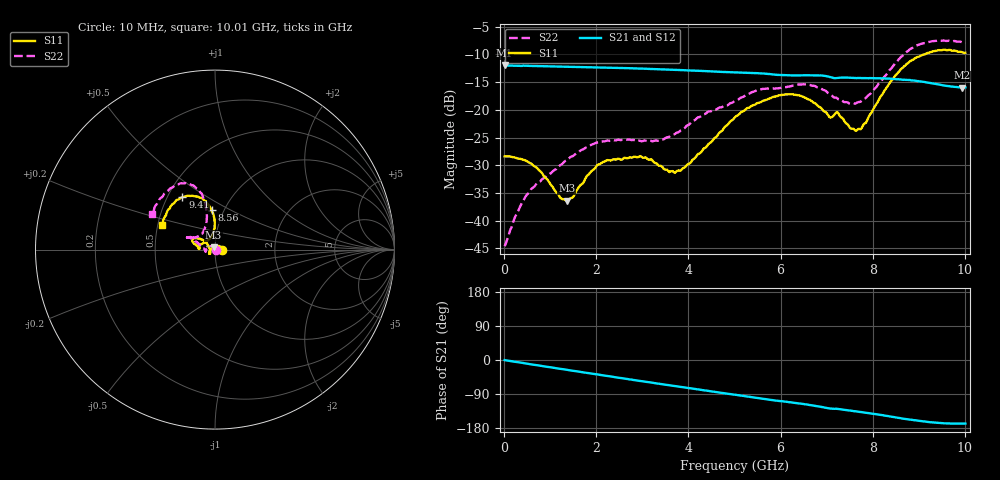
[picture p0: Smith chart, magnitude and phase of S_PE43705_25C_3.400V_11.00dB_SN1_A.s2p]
! Device ID: PE43705
! Serial: 1
! Insertion: A
! Impedance: 50 ohm
! Temp: 25C
! VDD: 3.400V
! Attenuation Step: 11.00dB
#  Hz  S  RI  R  50
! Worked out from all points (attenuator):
!   401 points, 10 MHz to 10.01 GHz, reference 50 ohm
!   highest |S21| = -12.00 dB at 10 MHz (marker M1); lowest = -16.0 dB at 9.935 GHz (marker M2)
!   lowest |S11| = -36.4 dB at 1.36 GHz (marker M3), VSWR 1.03, Z = 49.2 + j1.28 ohm
!   |S11| at or under -10 dB: start of sweep to 9.117 GHz
!   |S22| runs from -44.6 to -7.5 dB; largest |S21 - S12| = 0.002
!   S11 on the Smith chart (normalised r, x): 10 MHz: 1.08, +0.00; 8.56 GHz: 0.88, +0.40; 9.41 GHz: 0.60, +0.40; 10.01 GHz: 0.52, +0.16
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1e7  0.038 0.000161  0.2511 -0.00112  0.2514 -0.00107  0.00587 0.000351
2.85e8  0.0351 0.00959  0.2484 -0.0244  0.2484 -0.0242  0.00481 0.0108
5.1e8  0.0296 0.0167  0.2453 -0.0433  0.2454 -0.0431  0.000419 0.0175
1.36e9  -0.00792 0.013  0.2207 -0.1072  0.2207 -0.107  -0.0318 0.0149
1.685e9  -0.0211 0.00302  0.2067 -0.1288  0.2068 -0.1287  -0.043 0.00696
2.21e9  -0.0315 -0.0148  0.1798 -0.1599  0.1799 -0.1598  -0.0521 -0.00646
2.96e9  -0.03 -0.0237  0.1335 -0.1941  0.1336 -0.1938  -0.0519 -0.00756
3.36e9  -0.0256 -0.018  0.1067 -0.2064  0.107 -0.2061  -0.0527 -0.00426
3.635e9  -0.0268 -0.00797  0.0879 -0.2127  0.0879 -0.2126  -0.0588 0.00163
3.86e9  -0.029 0.00254  0.0719 -0.2165  0.072 -0.2164  -0.0658 0.00907
5.01e9  -0.0667 0.054  -0.0065 -0.2173  -0.00626 -0.2174  -0.111 0.0476
5.985e9  -0.1208 0.0617  -0.0646 -0.1959  -0.0637 -0.1958  -0.1421 0.0672
6.685e9  -0.1144 0.031  -0.1017 -0.1776  -0.1017 -0.1776  -0.1507 0.0673
7.06e9  -0.0852 0.0119  -0.1214 -0.1564  -0.1211 -0.157  -0.1204 0.0694
7.335e9  -0.0794 0.0293  -0.1266 -0.1486  -0.1268 -0.1488  -0.0972 0.0729
7.685e9  -0.0366 0.0565  -0.1404 -0.1338  -0.1401 -0.1338  -0.0688 0.0952
8.36e9  -0.00333 0.173  -0.1634 -0.0994  -0.1626 -0.0999  -0.0481 0.2219
8.56e9  -0.0174 0.2185  -0.1685 -0.0858  -0.1669 -0.0866  -0.0593 0.2781
8.935e9  -0.0712 0.2864  -0.1716 -0.0639  -0.1708 -0.0627  -0.1221 0.3579
9.41e9  -0.1812 0.2927  -0.1646 -0.041  -0.1647 -0.041  -0.2216 0.3596
9.935e9  -0.2888 0.1633  -0.1551 -0.0338  -0.1558 -0.0343  -0.3391 0.2241
1.001e10  -0.2977 0.1358  -0.1558 -0.034  -0.1561 -0.0348  -0.3534 0.196
